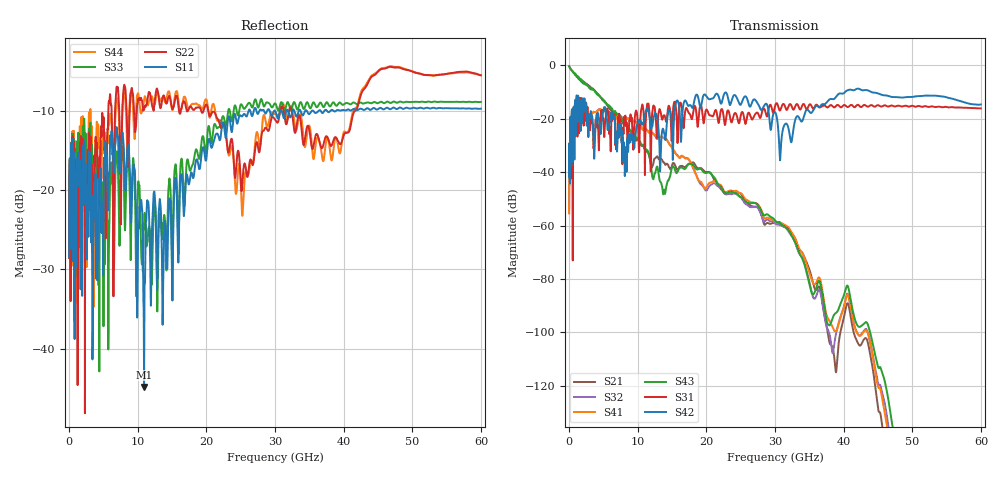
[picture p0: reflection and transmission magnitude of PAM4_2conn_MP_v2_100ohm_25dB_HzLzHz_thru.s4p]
! Info: Touchstone file created by Circ.  Input file=FAB50GbE_2conn_Midplane_Examax_Topo2_v2_100ohm_25dB_HzLzHz.circ
# Hz S RI R 50
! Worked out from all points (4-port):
!   6000 points, 10 MHz to 60 GHz, reference 50 ohm
!   strongest paths, dB at 10 MHz, 15.01 GHz, 30.01 GHz, 45.01 GHz, 60 GHz:
!     S42: -41.6, -24.7, -17.5, -10.5, -14.7
!     S31: -41.7, -24.1, -15.3, -14.9, -16.1
!     S43: -0.3, -38.1, -58.1, -112.9, -172.8
!     S41: -55.4, -30.7, -58.4, -120.2, -180.8
!     S32: -55.4, -30.9, -59.0, -118.9, -179.0
!     S21: -0.3, -37.5, -59.3, -128.5, -188.6
!   lowest |S11| = -44.8 dB at 10.93 GHz (marker M1), VSWR 1.01, Z = 50.1 - j0.562 ohm
!   |S11| at or under -10 dB: start of sweep to 26.15 GHz; 34.61 GHz to 35.41 GHz (794.7 MHz wide, 2.27 % of centre); 35.54 GHz to 36.4 GHz (862.3 MHz wide, 2.4 % of centre)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
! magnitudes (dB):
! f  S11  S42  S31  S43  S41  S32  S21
! 10 MHz  -28.5  -41.6  -41.7  -0.3  -55.4  -55.4  -0.3
! 1.3 GHz  -16.0  -11.7  -13.5  -4.8  -18.0  -18.1  -4.6
! 8.14 GHz  -18.9  -40.8  -21.1  -21.9  -20.3  -20.5  -22.6
! 10.93 GHz  -44.8  -20.1  -21.6  -30.6  -23.9  -23.7  -31.0
! 27.31 GHz  -10.1  -13.6  -17.8  -51.8  -51.7  -53.1  -52.8
! 35.16 GHz  -10.3  -17.8  -14.6  -83.5  -78.9  -82.6  -77.7
! 60 GHz  -9.8  -14.7  -16.1  -172.8  -180.8  -179.0  -188.6
